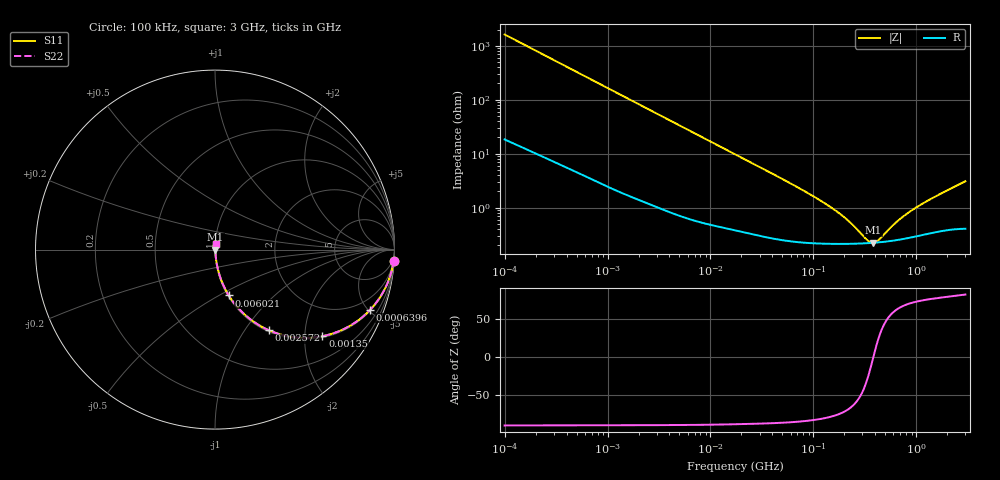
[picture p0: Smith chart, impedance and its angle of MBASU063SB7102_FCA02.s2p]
! MBASU063SB7102_FCA02  S-PARAMETER MODEL  ( Standard Model )
! Model Generated by TAIYO YUDEN Corporation (https://www.yuden.co.jp/en/)
! Version 1.0
! TAIYO YUDEN Control No. 250312
! Copyright(c) 2025 TAIYO YUDEN CO.,LTD. All Rights Reserved.
! Product Description (link to TY-COMPAS)
! https://ds.yuden.co.jp/TYCOMPAS/or/detail?pn=MBASU063SB7102KFCA02&u=M
! Products Name : Multilayer Ceramic Capacitors
! Characteristics :
!  Capacitance : 1000 [pF] , Rated Voltage : 50 [V] , TCC : X7R
!  Case Size : 0.6 x 0.3 / 0.024 x 0.012 [mm/inch] , Thickness : 0.3 / 0.012 [mm/inch]
!  (Conditions: Temperature = 25 [degC] , DC Bias Voltage = 0 [V])
! External Node Assignments :
!  1  o---| |---o  2
! GND o---------o GND
! Frequency Range : 100kHz  -  3GHz  [ 401 STEP ]
# MHZ S RI R 50
! Freq[MHz].  S11 Real  S11 Imag  S21 Real  S21 Imag  S12 Real  S12 Imag  S22 Real  S22 Imag
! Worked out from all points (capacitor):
!   401 points, 100 kHz to 3 GHz, reference 50 ohm
!   read as one part in series: C = 981 pF near 105.3 kHz
!   lowest |Z| = 223 mohm at 381.7 MHz (marker M1)
!   series resonance near 381.8 MHz, so ESL is about 180 pH
!   S11 on the Smith chart (normalised r, x): 100 kHz: 1, -32; 639.6 kHz: 1.07, -5.14; 1.35 MHz: 1.04, -2.45; 2.572 MHz: 1.02, -1.29; 6.021 MHz: 1.01, -0.56; 3 GHz: 1.01, +0.06
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0.1  0.9955 -0.0614  0.00449 0.0614  0.00449 0.0614  0.9955 -0.0614
0.246461  0.9759 -0.1472  0.0241 0.1472  0.0241 0.1472  0.9759 -0.1472
0.562235  0.8917 -0.3038  0.1083 0.3038  0.1083 0.3038  0.8917 -0.3038
0.639561  0.8651 -0.3346  0.1349 0.3346  0.1349 0.3346  0.8651 -0.3346
0.917447  0.7604 -0.4196  0.2396 0.4196  0.2396 0.4196  0.7604 -0.4196
1.350433  0.5987 -0.4825  0.4013 0.4825  0.4013 0.4825  0.5987 -0.4825
1.839868  0.4493 -0.4892  0.5507 0.4892  0.5507 0.4892  0.4493 -0.4892
2.572132  0.2984 -0.4487  0.7016 0.4487  0.7016 0.4487  0.2984 -0.4487
3.161081  0.222 -0.4064  0.778 0.4064  0.778 0.4064  0.222 -0.4064
6.020821  0.0769 -0.2555  0.9231 0.2555  0.9231 0.2555  0.0769 -0.2555
10.08119  0.0315 -0.161  0.9685 0.161  0.9685 0.161  0.0315 -0.161
17.7727  0.0126 -0.0937  0.9874 0.0937  0.9874 0.0937  0.0126 -0.0937
97.38194  0.00246 -0.0165  0.9975 0.0165  0.9975 0.0165  0.00246 -0.0165
180.7614  0.00217 -0.00738  0.9978 0.00738  0.9978 0.00738  0.00217 -0.00738
233.9019  0.00215 -0.00459  0.9978 0.00459  0.9978 0.00459  0.00215 -0.00459
335.5313  0.00219 -0.00116  0.9978 0.00116  0.9978 0.00116  0.00219 -0.00116
381.6779  0.00222 -2.65e-06  0.9978 2.65e-06  0.9978 2.65e-06  0.00222 -2.65e-06
434.1712  0.00227 0.00115  0.9977 -0.00115  0.9977 -0.00115  0.00227 0.00115
547.5153  0.00239 0.00326  0.9976 -0.00326  0.9976 -0.00326  0.00239 0.00326
726.971  0.00263 0.00604  0.9974 -0.00604  0.9974 -0.00604  0.00263 0.00604
1016.304  0.00304 0.0098  0.997 -0.0098  0.997 -0.0098  0.00304 0.0098
3000  0.00497 0.0304  0.995 -0.0304  0.995 -0.0304  0.00497 0.0304
